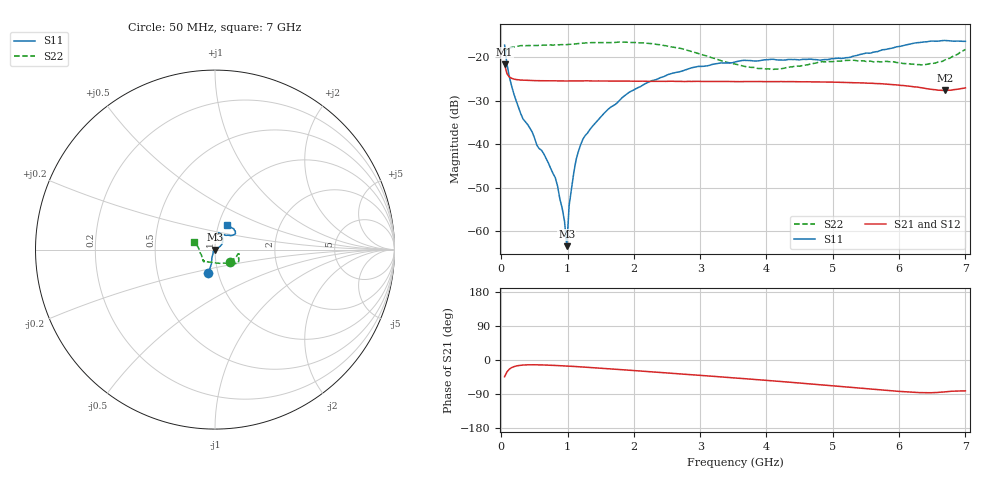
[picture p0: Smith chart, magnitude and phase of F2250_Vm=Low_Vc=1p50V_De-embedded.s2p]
! Integrated Device Technology
! Corporate Headquarters
! 6024 Silver Creek Valley Road
! San Jose, CA 95138  USA
! Phone:  1-408-284-8200
! Toll Free:  1-800-223-1366
! Webpage:  http://www.idt.com/
! Timing and RF Division
! 515 Groton Road, Suite 102
! Westford, MA 01886-6024
! Device:  F2250
! Description: Voltage Variable RF Attenuator
! Frequency:  50.0 -  6000.00 MHz
! Package:  3x3 mm Thin QFN Plastic Package: 16 pin
! Ports:  2 RF, 3 DC
!  Pin  1  = GND
!  Pin  2  = NC
!  Pin  3  = RF1  = Port 1
!  Pin  4  = NC
!  Pin  5  = GND
!  Pin  6  = GND
!  Pin  7  = GND
!  Pin  8  = GND
!  Pin  9  = NC
!  Pin 10  = RF2  = Port 2
!  Pin 11  = NC
!  Pin 12  = GND
!  Pin 13  = GND
!  Pin 14  = VCNTRL
!  Pin 15  = VDD
!  Pin 16  = VMODE
! Vcntrl:  1.500 Volts
! Vmode:  +0.000 Volts
! Vdd:  +3.30  Volts
! Current:  1.191 mA
! Data:  The device was measured on a the F2250 evaluation board which has
!  individual transmission lines to the RF pins.  Data was collected
!  using a calibrated network analyzer.  The evaluation board was
!  de-embedded using a TRL calibration technique.
!  The reference plane is the edge of the package pin.
! Misc:  SN 10
!  Action Tracker AT0258
! Date Measured:  2014-11-26
! Date:  2015-10-15  MJV
! Note:
!  Integrated Device Technology supplies this data as a sample of measured
!  data at the package pin for this product.  Your particular data for this
!  product may vary.
!  Data was taken at 25 degrees C.
!  Integrated Device Technology reserves the right to change this data at anytime.
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# GHz S dB R 50
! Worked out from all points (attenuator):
!   201 points, 50 MHz to 7 GHz, reference 50 ohm
!   highest |S21| = -21.69 dB at 50 MHz (marker M1); lowest = -27.7 dB at 6.687 GHz (marker M2)
!   lowest |S11| = -63.5 dB at 988.2 MHz (marker M3), VSWR 1.00, Z = 50.1 - j0.0201 ohm
!   |S11| at or under -10 dB: start of sweep to end of sweep
!   |S22| runs from -22.8 to -16.5 dB; largest |S21 - S12| = 0.00025
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0.05  -17.23 -106.2  -21.69 -44.1  -21.70 -44.1  -19.24 -39.6
0.08475  -21.55 -104.0  -23.77 -31.5  -23.79 -31.5  -18.08 -19.7
0.1195  -24.39 -107.3  -24.53 -24.4  -24.54 -24.4  -17.87 -13.7
0.29325  -32.99 -117.0  -25.27 -13.9  -25.28 -13.9  -17.35 -10.4
0.8145  -47.72 -177.6  -25.45 -14.4  -25.45 -14.4  -17.19 -17.0
0.9535  -57.73 -158.2  -25.48 -15.6  -25.48 -15.6  -17.18 -19.5
0.98825  -63.46 -17.4  -25.48 -15.9  -25.48 -15.9  -17.12 -19.9
1.023  -54.13 6.4  -25.47 -16.2  -25.48 -16.2  -17.06 -20.0
1.0925  -46.64 16.4  -25.48 -16.9  -25.47 -16.9  -17.00 -21.1
1.12725  -43.64 19.7  -25.47 -17.3  -25.46 -17.3  -16.92 -21.8
1.2315  -38.83 21.7  -25.46 -18.5  -25.46 -18.5  -16.77 -23.6
1.5095  -33.55 28.2  -25.49 -21.8  -25.49 -21.8  -16.66 -26.1
1.857  -28.90 33.4  -25.52 -26.1  -25.52 -26.0  -16.53 -29.5
2.37825  -24.86 42.7  -25.56 -32.5  -25.53 -32.5  -17.11 -34.0
2.93425  -22.23 56.8  -25.57 -39.6  -25.55 -39.6  -18.99 -42.6
3.525  -21.12 70.4  -25.61 -47.4  -25.62 -47.4  -21.57 -67.5
4.081  -20.48 77.7  -25.62 -54.9  -25.61 -54.9  -22.80 -100.4
4.7065  -20.54 71.2  -25.69 -63.8  -25.68 -63.8  -21.47 -125.5
5.85325  -18.04 39.3  -26.23 -80.8  -26.23 -80.8  -21.06 -139.9
6.3745  -16.50 40.6  -27.14 -86.3  -27.13 -86.3  -21.76 -160.4
6.68725  -16.16 48.1  -27.66 -84.2  -27.65 -84.2  -20.66 174.1
7  -16.36 62.8  -27.05 -81.4  -27.05 -81.4  -18.23 160.6
